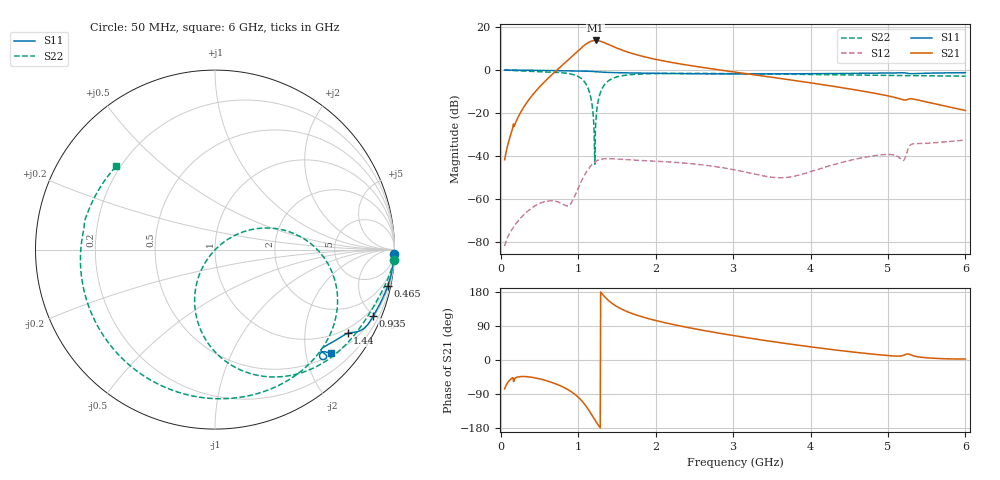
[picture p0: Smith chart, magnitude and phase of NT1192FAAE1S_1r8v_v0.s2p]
! Created Fri May 20 14:16:06 2022
# hz S ma R 50
! 2 Port Network Data from SP10.SP block
! freq  magS11  angS11  magS21  angS21  magS12  angS12  magS22  angS22
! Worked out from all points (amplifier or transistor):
!   1191 points, 50 MHz to 6 GHz, reference 50 ohm
!   highest |S21| = 13.7 dB at 1.225 GHz (marker M1)
!   |S21| within 3 dB of that: 1.055 GHz to 1.464 GHz (408.4 MHz wide, 32.4 % of centre)
!   unconditionally stable (mu >= 1): start of sweep to end of sweep
!   at 1.04 GHz: K = 4.05, MAG = 22.0 dB, |S12| = -51.8 dB
!   at 3.025 GHz: K = 13.24, MAG = 8.5 dB, |S12| = -46.4 dB
!   at 6 GHz: K = 22.15, MAG = -9.6 dB, |S12| = -32.6 dB
!   lowest NFmin = 0.50 dB at 815 MHz
!   S11 on the Smith chart (normalised r, x): 50 MHz: 8, -86; 465 MHz: 0.76, -9.50; 935 MHz: 0.57, -4.90; 1.44 GHz: 0.83, -3.26; 6 GHz: 0.54, -2.52
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5e7  0.9978 -1.3  0.008187 -76.3  8.048e-05 113.1  0.9967 -3.4
1.75e8  0.9958 -4.6  0.04965 -51.9  0.0002416 103.2  0.9711 -11.0
4.65e8  0.9835 -11.9  0.3431 -48.0  0.000733 97.7  0.9224 -26.1
7.3e8  0.9674 -18.2  1.014 -64.6  0.0008696 96.7  0.8818 -43.3
9.35e8  0.9563 -22.8  2.199 -87.2  0.0009836 165.6  0.7837 -64.9
1.045e9  0.9501 -25.5  3.324 -107.4  0.002681 179.4  0.6236 -84.7
1.095e9  0.9449 -26.8  3.932 -120.1  0.003954 173.4  0.4902 -97.1
1.135e9  0.9382 -28.0  4.382 -131.8  0.005124 165.4  0.3469 -108.7
1.2e9  0.9218 -29.6  4.832 -153.0  0.006944 148.6  0.06206 -128.7
1.225e9  0.9145 -30.0  4.869 -161.1  0.007498 141.7  0.05125 40.9
1.265e9  0.9033 -30.6  4.779 -173.4  0.008141 131.2  0.2187 29.7
1.33e9  0.8886 -31.3  4.385 169.5  0.008625 116.5  0.4306 13.1
1.44e9  0.8735 -32.3  3.596 149.0  0.008643 99.2  0.6335 -7.1
1.55e9  0.8642 -33.3  2.983 135.4  0.008427 88.0  0.7279 -20.5
1.68e9  0.8553 -34.6  2.48 123.8  0.008201 79.0  0.7817 -31.9
2.035e9  0.8362 -37.7  1.72 102.5  0.007547 62.1  0.8287 -53.6
3.025e9  0.8118 -42.6  0.894 63.8  0.00477 19.2  0.8252 -98.3
4.02e9  0.8215 -43.8  0.4981 34.2  0.004445 -96.2  0.7869 -140.5
5.01e9  0.8538 -43.5  0.2487 11.5  0.01091 -147.1  0.7462 178.4
5.195e9  0.8649 -45.0  0.2031 11.9  0.007918 -132.0  0.7396 171.3
5.32e9  0.8257 -43.8  0.2128 11.6  0.01917 -130.8  0.7417 166.1
6e9  0.868 -41.8  0.1145 2.7  0.02354 -163.6  0.7201 140.0
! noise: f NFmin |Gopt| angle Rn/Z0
5e+07  2.978  0.9925  1.349  101.5
7.1e+08  0.5118  0.8703  15.48  0.7919
1.37e+09  0.6356  0.8073  26.25  0.6374
2.03e+09  0.9439  0.779  35.58  0.7563
2.69e+09  1.377  0.7681  41.95  0.9761
3.355e+09  2.031  0.7696  45.27  1.398
4.015e+09  3.06  0.7812  45.96  2.303
4.675e+09  4.707  0.8047  44.99  4.612
5.335e+09  7.365  0.8071  44.47  9.859
6e+09  10.88  0.8536  41.93  32.66
